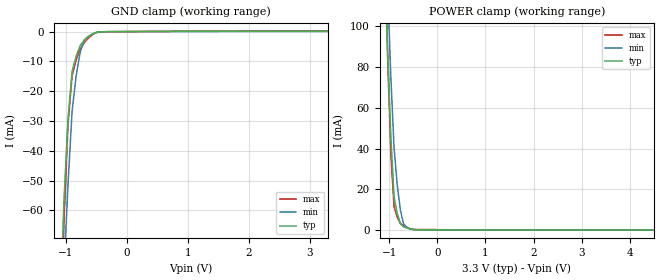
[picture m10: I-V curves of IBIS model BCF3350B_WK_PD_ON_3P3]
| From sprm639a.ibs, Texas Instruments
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|   Model Cell BCF3350B_WK_PD_ON_3P3
|BCF3350B_WK_PD_ON_3P3
[Model]   BCF3350B_WK_PD_ON_3P3
Model_type   Input
Polarity   Non-Inverting
Vinl =  0.8
Vinh =  2
C_comp   1.081689p   0.9467568p   1.2214p
[Model Spec]
Vinl   0.8   0.8   0.8
Vinh   2   2   2
[Temperature Range]   25   155   -40
[Voltage Range]   3.3   2.97   3.63
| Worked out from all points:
|   GND clamp passes 1 mA (typ) near -0.58 V on its own axis
|   POWER clamp passes 1 mA (typ) near -0.64 V on its own axis
| Nom Voltages:
|   VDD=1.2, VDDS=3.3, VSS=0
| Min Voltages:
|   VDD=1.08, VDDS=2.97, VSS=0
| Max Voltages:
|   VDD=1.32, VDDS=3.63, VSS=0
[POWER_clamp]
|   voltage   I(typ)   I(min)   I(max)
-3.3V     2.318A     2.595A     3.049A
-1.1V     141.5mA    168mA      152.4mA
-1.033V   87.22mA    117.8mA    84.5mA
-966.7mV  45.46mA    75.19mA    37.47mA
-900mV    16.26mA    40.27mA    11.33mA
-833.3mV  7.927mA    21.99mA    6.203mA
-766.7mV  3.013mA    9.498mA    3.099mA
-700mV    1.521mA    2.801mA    2.021mA
-566.7mV  472.3uA    527.3uA    648.9uA
-366.7mV  111.4uA    66.02uA    181.9uA
6.6V      0A         0A         0A
[GND_clamp]
|   voltage   I(typ)   I(min)   I(max)
-3.3V     -1.888A    -1.585A    -3.154A
-1.1V     -95.79mA   -113.9mA   -112.1mA
-1.033V   -56.71mA   -80.31mA   -63.62mA
-966.7mV  -29.26mA   -51.23mA   -31.17mA
-900mV    -13.43mA   -26.68mA   -14.76mA
-833.3mV  -8.27mA    -14.79mA   -9.517mA
-766.7mV  -4.725mA   -6.876mA   -5.842mA
-700mV    -2.797mA   -2.931mA   -3.733mA
-566.7mV  -794.1uA   -808.3uA   -1.042mA
-500mV    -234.8uA   -305.8uA   -282.8uA
-366.7mV  -42.38uA   -46.42uA   -57.66uA
3.3V      107.2uA    55.45uA    177.9uA
